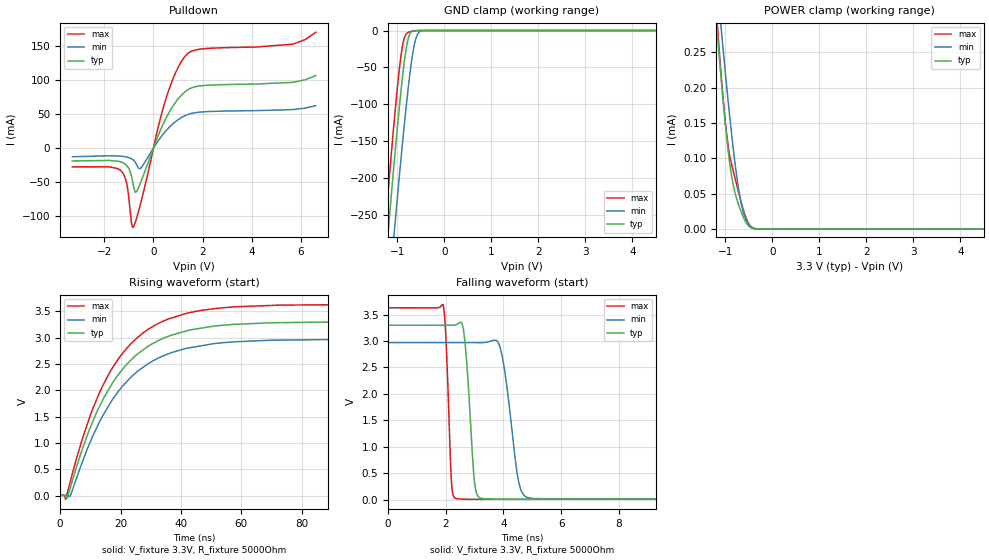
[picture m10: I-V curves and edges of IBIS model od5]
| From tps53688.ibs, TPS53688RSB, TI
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|   od5 Model
[Model]   od5
Model_type   Open_drain
Polarity   Non-Inverting
Vmeas = 1.65
Vref = 3.3
Cref = 2pF
Rref = 5000
|   typ   min   max
C_comp   1.505pF   1.485pF   1.533pF
[Voltage Range]   3.3   2.97   3.63
|Junction Temperature
[Temperature Range]   25   125   -40
[Pullup Reference]   3.3   2.97   3.63
[Pulldown Reference]   -0   -0   -0
[Power Clamp Reference]   3.3   2.97   3.63
[GND Clamp Reference]   0   0   0
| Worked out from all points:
|   slope of the pulldown table from 0 to 0.495 V, typ, clamps not added: 11.5 ohm
|   GND clamp passes 1 mA (typ) near -0.68 V on its own axis
|   POWER clamp passes 1 mA (typ) near -2.01 V on its own axis
|   falling waveform, V_fixture 3.3V, R_fixture 5000Ohm: 20-80 % time 227ps typ, 389ps min, 146ps max; typ from 3.3 V to 0.006 V
|   rising waveform, V_fixture 3.3V, R_fixture 5000Ohm: 20-80 % time 18.6ns typ, 18.9ns min, 18.2ns max; typ from 0.006 V to 3.3 V
[Pulldown]
|   Voltage   I(typ)   I(min)   I(max)
-3.3V     -18.98mA   -12.81mA   -27.69mA
-1.31V    -20.63mA   -11.99mA   -33.74mA
-1.092V   -25.6mA    -13.25mA   -51.31mA
-894.3mV  -40.91mA   -15.8mA    -110.3mA
-815.1mV  -55.91mA   -17.76mA   -116.5mA
-745.8mV  -65.32mA   -20.65mA   -110.2mA
-528mV    -51.15mA   -30.1mA    -82.25mA
491.7mV   42.67mA    24.74mA    70.84mA
917.4mV   68.37mA    39.51mA    112.5mA
1.353V    84.82mA    48.79mA    137.8mA
5.669V    96.77mA    56.65mA    153mA
6.6V      106.7mA    62.42mA    170.5mA
[GND Clamp]
|   Voltage   I(typ)   I(min)   I(max)
-3.3V     -1.985A    -2.038A    -1.965A
-1.27V    -328.7mA   -423.3mA   -273.9mA
-1.181V   -260.7mA   -356.4mA   -204.8mA
-1.082V   -187.7mA   -283.8mA   -131.7mA
-1.023V   -145.9mA   -241.3mA   -90.9mA
-904.2mV  -69.32mA   -160mA     -24.98mA
-854.7mV  -42.42mA   -128mA     -9.948mA
-765.6mV  -9.625mA   -74.84mA   -2.42mA
-686.4mV  -1.183mA   -35.86mA   -859.6uA
-627mV    -260.9uA   -15.43mA   -300.2uA
-478.5mV  -8.563uA   -443.8uA   -10.22uA
6.6V      0A         0A         0A
[POWER Clamp]
|   Voltage   I(typ)   I(min)   I(max)
-3.3V     2.152mA    2.03mA     2.466mA
-1.241V   333.1uA    395.7uA    354.3uA
-1.132V   245.1uA    314.7uA    253.6uA
-1.092V   214.4uA    285.9uA    219.3uA
-1.003V   150uA      222.8uA    151.8uA
-933.9mV  106.8uA    176.1uA    114uA
-815.1mV  56.65uA    104uA      77.22uA
-735.9mV  37.78uA    64.34uA    56.41uA
-646.8mV  21.24uA    31.4uA     33.65uA
-547.8mV  7.883uA    11.36uA    13.62uA
-429mV    873nA      2.24uA     1.785uA
6.6V      0A         0A         0A
[Ramp]
R_load = 5000
|   typ   min   max
dV/dt_r   1.97612/1.86038e-08   1.77598/1.89264e-08   2.17546/1.82381e-08
dV/dt_f   1.97612/2.25908e-10   1.77598/3.8871e-10   2.17546/1.45714e-10
[Falling Waveform]
V_fixture = 3.3V
V_fixture_min = 2.97V
V_fixture_max = 3.63V
R_fixture = 5000Ohm
C_fixture = 0F
|   Time   V(typ)   V(min)   V(max)
0s        3.3V       2.97V      3.63V
1.903ns   3.298V     2.969V     3.686V
2.224ns   3.298V     2.969V     173.2mV
2.57ns    3.32V      2.969V     8.818mV
2.74ns    2.485V     2.968V     5.509mV
3.098ns   77.72mV    2.968V     5.508mV
3.891ns   8.314mV    2.864V     5.506mV
4.641ns   8.311mV    137.9mV    5.504mV
5.585ns   8.307mV    12.84mV    5.502mV
500ns     6.465mV    10.03mV    4.231mV
[Rising Waveform]
V_fixture = 3.3V
V_fixture_min = 2.97V
V_fixture_max = 3.63V
R_fixture = 5000Ohm
C_fixture = 0F
|   Time   V(typ)   V(min)   V(max)
0s        6.465mV    10.03mV    4.231mV
1.815ns   -5.119mV   10.46mV    -69.86mV
2.315ns   -47.05mV   6.78mV     37.02mV
3.329ns   143.2mV    -6.218mV   258.8mV
11.02ns   1.437V     1.158V     1.68V
16.06ns   2.013V     1.706V     2.303V
20.6ns    2.394V     2.075V     2.699V
33.44ns   2.969V     2.636V     3.296V
51.33ns   3.222V     2.889V     3.553V
500ns     3.3V       2.97V      3.63V
